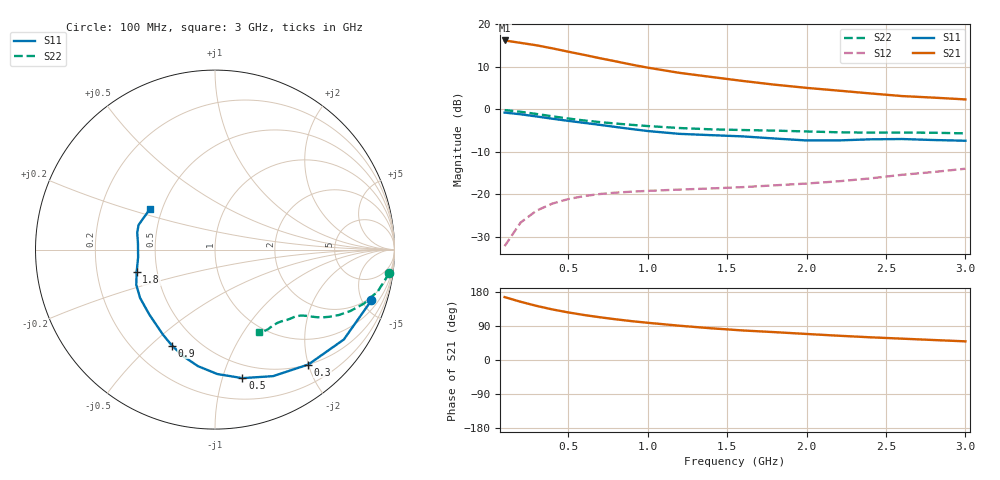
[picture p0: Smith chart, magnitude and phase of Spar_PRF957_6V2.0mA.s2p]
! Filename:  PRF957L.S2P  Version:  3.0
! NXP part #:  PRF957  Date:  Nov 1998
! Bias condition:  Vce=6V, Ic=2mA
#  MHz  S  MA  R 50
! Freq  S11  S21  S12  S22
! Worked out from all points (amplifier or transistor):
!   20 points, 100 MHz to 3 GHz, reference 50 ohm
!   highest |S21| = 16.2 dB at 100 MHz (marker M1)
!   |S21| within 3 dB of that: start of sweep to 548.1 MHz
!   unconditionally stable (mu >= 1): 1.837 GHz to end of sweep
!   at 400 MHz: K = 0.24, MSG = 18.3 dB, |S12| = -22.2 dB
!   at 1.2 GHz: K = 0.72, MSG = 13.7 dB, |S12| = -18.9 dB
!   at 3 GHz: K = 1.09, MAG = 6.3 dB, |S12| = -14.0 dB
!   lowest NFmin = 0.93 dB at 500 MHz
!   S11 on the Smith chart (normalised r, x): 100 MHz: 1.66, -5.86; 300 MHz: 0.50, -2.00; 500 MHz: 0.38, -1.16; 900 MHz: 0.36, -0.59; 1.8 GHz: 0.38, -0.12; 3 GHz: 0.43, +0.24
100  0.9163 -18.0  6.464 166.0  0.02455 79.6  0.9799 -7.6
200  0.8753 -34.9  6.058 153.7  0.04641 70.7  0.9366 -14.4
300  0.8248 -51.0  5.672 142.9  0.06418 63.3  0.8829 -19.9
400  0.7756 -65.4  5.22 133.5  0.07776 57.5  0.8287 -24.4
500  0.7322 -78.0  4.772 125.6  0.08786 53.3  0.7804 -27.9
600  0.6932 -89.0  4.374 118.7  0.09541 50.1  0.7399 -30.4
700  0.6564 -98.3  3.995 112.8  0.1009 48.0  0.7077 -32.2
800  0.6199 -106.6  3.668 107.4  0.1047 46.5  0.6805 -33.6
900  0.5861 -114.1  3.357 102.5  0.1074 45.8  0.6569 -34.6
1000  0.5558 -121.4  3.097 98.2  0.1098 45.7  0.6362 -35.6
1200  0.5146 -135.3  2.688 90.5  0.1137 46.3  0.6027 -37.5
1400  0.4969 -147.1  2.405 83.7  0.1173 47.9  0.5817 -39.9
1600  0.4804 -155.9  2.157 77.9  0.1216 51.1  0.5707 -42.2
1800  0.4535 -164.2  1.95 73.5  0.1276 54.8  0.5616 -44.2
2000  0.4304 -174.3  1.789 68.7  0.1339 58.6  0.5493 -46.2
2200  0.4307 175.3  1.661 64.1  0.1422 62.3  0.537 -49.3
2400  0.4438 167.6  1.54 59.9  0.1539 65.6  0.5318 -53.0
2600  0.4474 162.2  1.433 56.3  0.1696 68.7  0.533 -56.3
2800  0.4355 156.2  1.373 52.7  0.1832 71.5  0.5304 -59.1
3000  0.4271 148.0  1.309 49.2  0.2001 73.9  0.5213 -62.3
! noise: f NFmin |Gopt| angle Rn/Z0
500  0.93  0.48  39  0.25
800  1.05  0.46  43  0.28
900  1.1  0.48  65  0.26
1000  1.31  0.45  71  0.26
1500  1.34  0.44  112  0.22
2000  1.86  0.39  168  0.12
